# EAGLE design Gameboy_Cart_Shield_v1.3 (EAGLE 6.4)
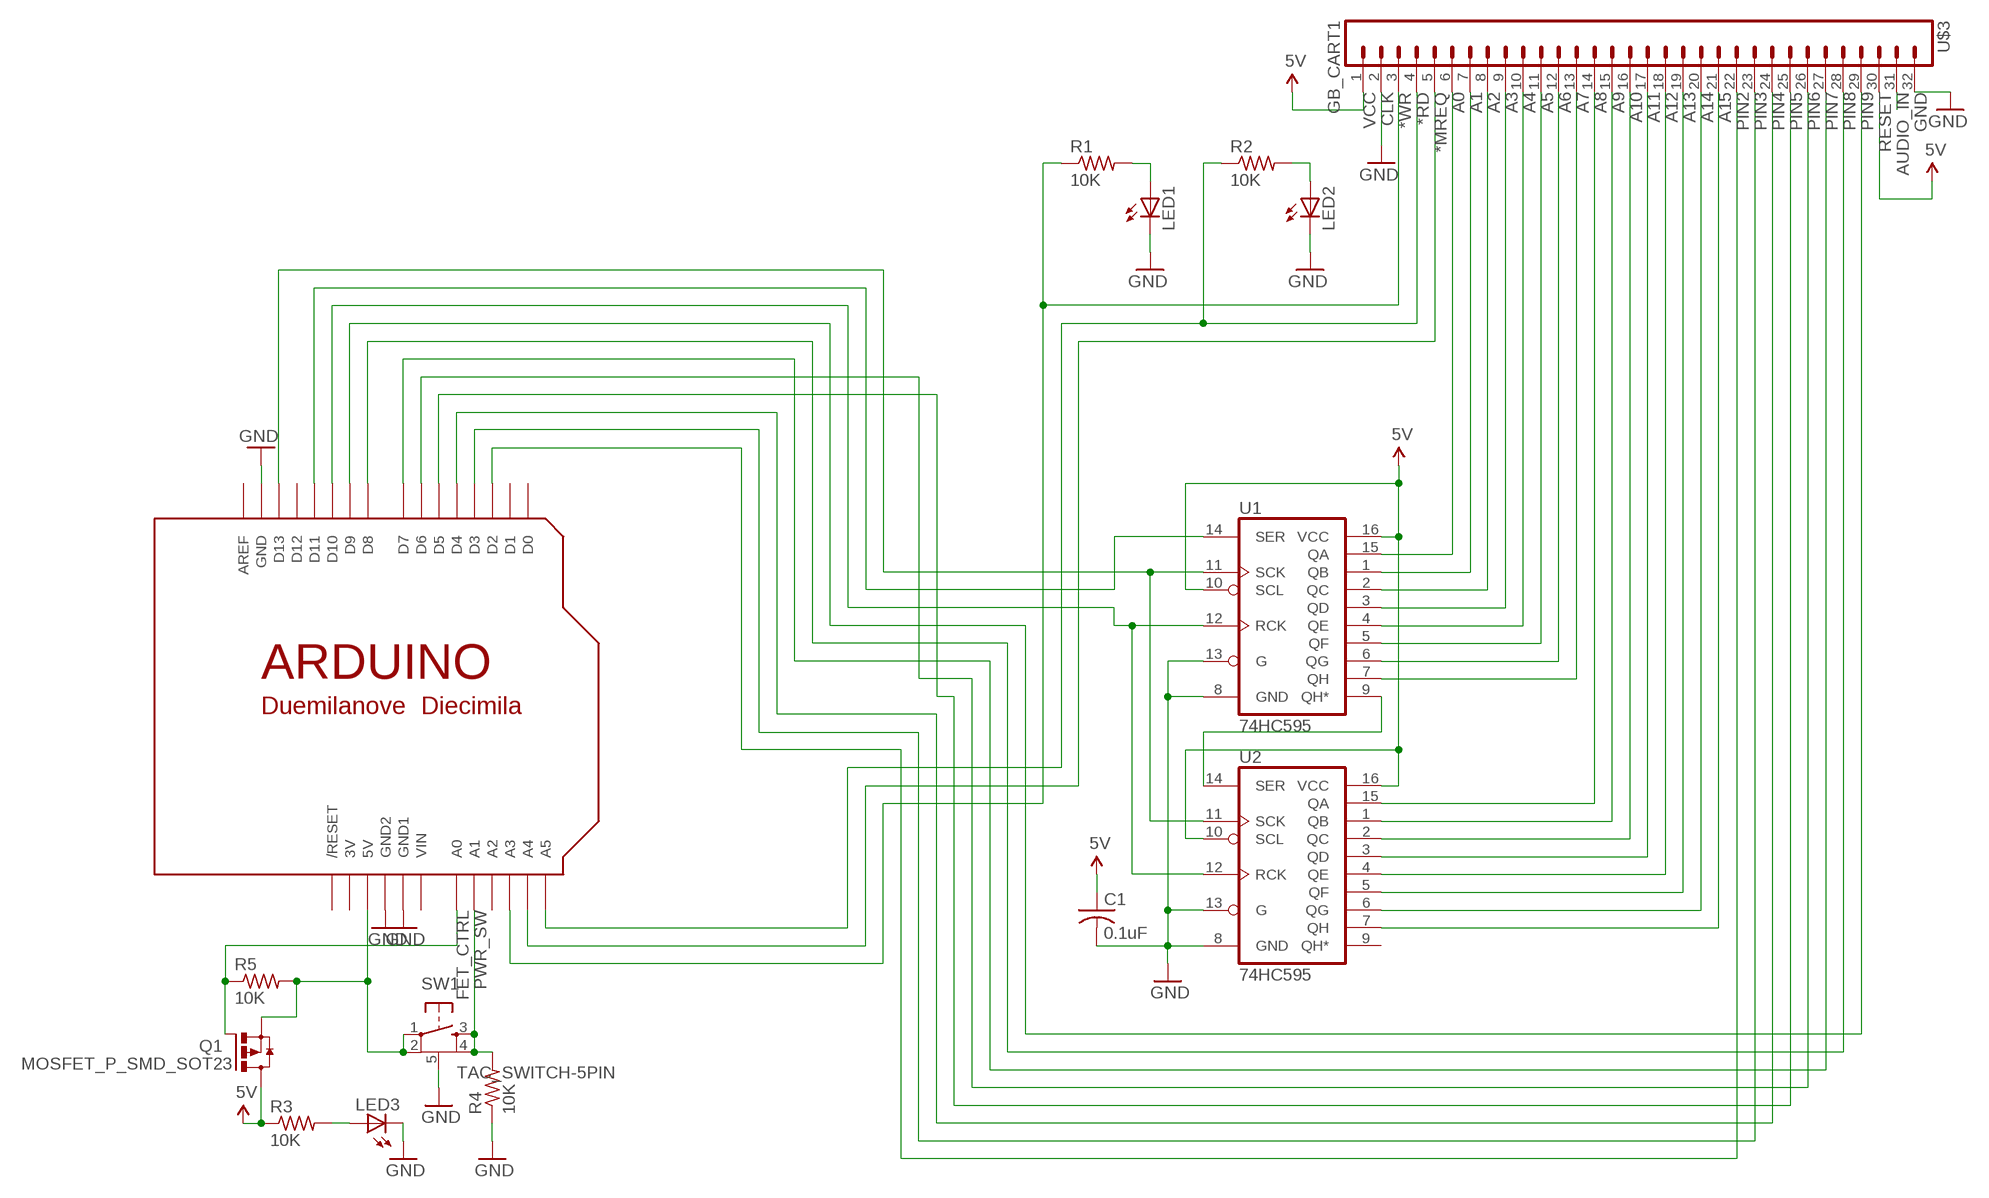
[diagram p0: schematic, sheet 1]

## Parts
C1  0.1uF  C-USC0805K  [C0805K]
LED1  LEDCHIP-LED0805  [CHIP-LED0805]
LED2  LEDCHIP-LED0805  [CHIP-LED0805]
LED3  LEDCHIP-LED0805  [CHIP-LED0805]
Q1  MOSFET_P_SMD_SOT23  [SUPER-SOT3]
R1  10K  R-US_R0805_2  [R0805_2]
R2  10K  R-US_R0805_2  [R0805_2]
R3  10K  R-US_R0805_2  [R0805_2]
R4  10K  R-US_R0805_2  [R0805_2]
R5  10K  R-US_R0805_2  [R0805_2]
SW1  TAC_SWITCH-5PIN  [TACTILE_SWITCH_SMD_6MM]
U1  74HC595  74LS595D  [SO16]
U2  74HC595  74LS595D  [SO16]
U$1  ARDUINONODIMA  [ARDUINO-NODIMA]
U$3  GB_CART1  [GB_CART_1]

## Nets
*MREQ: U$1.A4 U$3.5
*RD: R2.1 U$1.A5 U$3.4
*WR: R1.1 U$1.A3 U$3.3
A0: U1.15(QA) U$3.6
A1: U1.1(QB) U$3.7
A2: U1.2(QC) U$3.8
A3: U1.3(QD) U$3.9
A4: U1.4(QE) U$3.10
A5: U1.5(QF) U$3.11
A6: U1.6(QG) U$3.12
A7: U1.7(QH) U$3.13
A8: U2.15(QA) U$3.14
A9: U2.1(QB) U$3.15
A10: U2.2(QC) U$3.16
A11: U2.3(QD) U$3.17
A12: U2.4(QE) U$3.18
A13: U2.5(QF) U$3.19
A14: U2.6(QG) U$3.20
A15: U2.7(QH) U$3.21
AUDIO_IN: U$3.31
FET_CTRL: Q1.1(G) R5.1 U$1.A0
GND: C1.2 LED1.C LED2.C LED3.C R4.1 SW1.5 U1.8(GND) U1.13(G) U2.8(GND) U2.13(G) U$1.GND U$1.GND1 U$1.GND2 U$3.2 U$3.32
N$1: LED2.A R2.2
N$2: LED3.A R3.2
N$6: LED1.A R1.2
N$7: Q1.2(S) R5.2 SW1.1 SW1.2 U$1.5V
N$10: U1.9(QH*) U2.14(SER)
PIN2: U$1.D2 U$3.22
PIN3: U$1.D3 U$3.23
PIN4: U$1.D4 U$3.24
PIN5: U$1.D5 U$3.25
PIN6: U$1.D6 U$3.26
PIN7: U$1.D7 U$3.27
PIN8: U$1.D8 U$3.28
PIN9: U$1.D9 U$3.29
PIN10: U1.12(RCK) U2.12(RCK) U$1.D10
PIN11: U1.14(SER) U$1.D11
PIN12: U1.11(SCK) U2.11(SCK) U$1.D13
PWR_SW: R4.2 SW1.3 SW1.4 U$1.A1
VCC: C1.1 Q1.3(D) R3.1 U1.10(SCL) U1.16(VCC) U2.10(SCL) U2.16(VCC) U$3.1 U$3.30 ; supply symbol labelled 5V
Unconnected: U2.9(QH*) U$1.A2 U$1.AREF U$1.D0 U$1.D1 U$1.D12 U$1.RESET(/RESET)

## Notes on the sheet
- VCC | CLK | RESET

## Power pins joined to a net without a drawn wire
3V: U$1.3V
VIN: U$1.VIN

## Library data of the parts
C1 = adafruit:C-US: CAPACITOR, American symbol
LED1-LED3 = adafruit:LED: LED
Q1 = transistor-power_old:MOSFET_P_SMD_SOT23
R1-R5 = adafruit:R-US_: RESISTOR, American symbol
SW1 = SparkFun:TAC_SWITCH-5PIN
U1 U2 = SparkFun:74*595: 8-bit SHIFT REGISTER, output latch
U$1 = adafruit:ARDUINO: Arduino Diecimila/Duemilanove Make a shield with ease, this package has all the named pins as well as the two mounting drill holes and an outline of the USB and DC power connector. The outline is on the DIMENSION layer, so if your board house uses it they will cut the outline to match.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
U$3 = alex:GB_CART

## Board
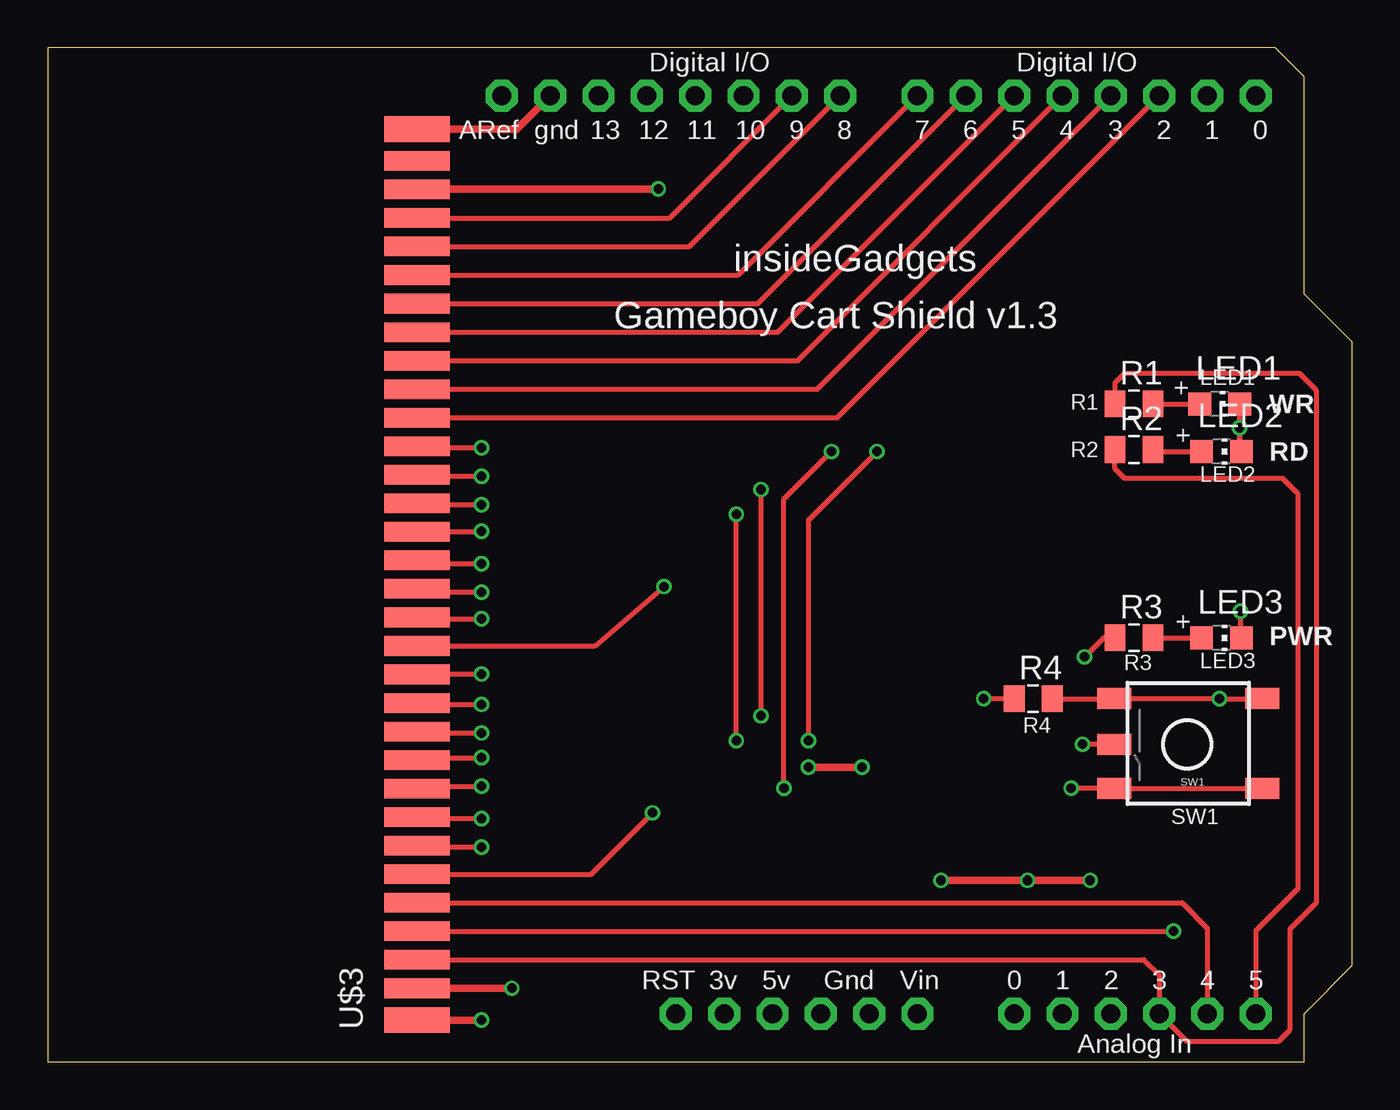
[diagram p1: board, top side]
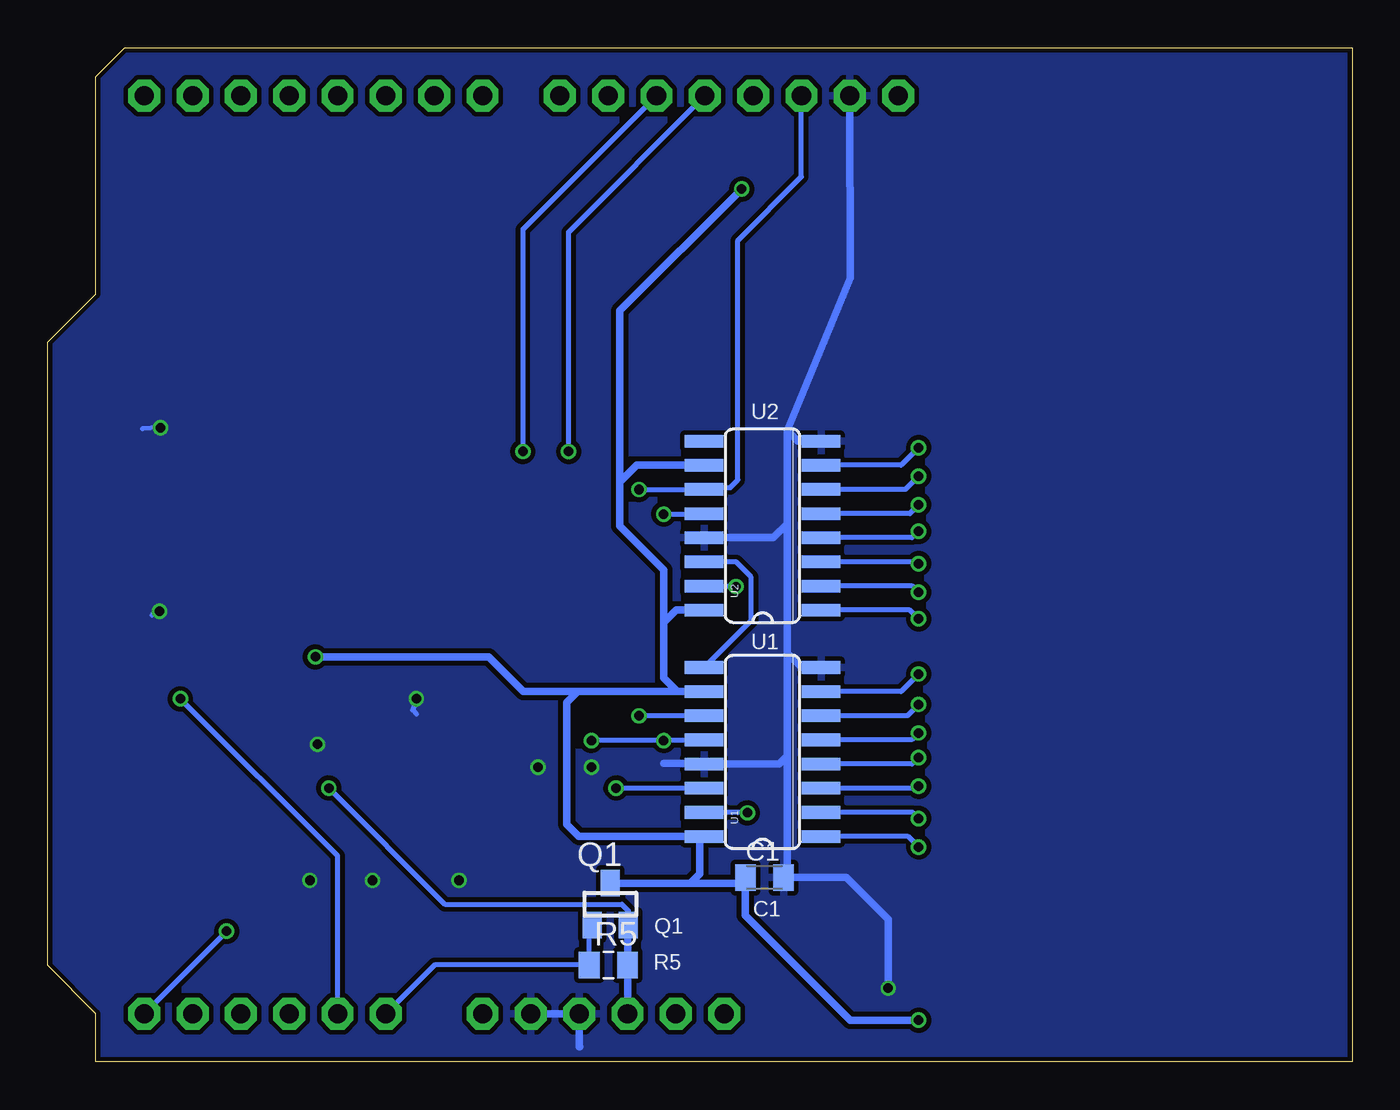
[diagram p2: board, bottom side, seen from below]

Size 68.58 x 53.34 mm. Coordinates in mm from the lower left corner, seen from the top.
Copper layers (1*16): Top 0.035mm / dielectric 1.5mm / Bottom 0.035mm
Design rules "ITEADstudio_DRC": minimum track width 6mil, minimum drill 12mil, track to track 6mil, track to pad 6mil, pad to pad 6mil, via to via 6mil, smd to smd 0mil, copper to edge 10mil, drill to drill 10mil, minimum pad ring 10mil, minimum via ring 6mil, stop-mask expansion 2mil, vias tented up to drill 100mil, thermal gap 10mil

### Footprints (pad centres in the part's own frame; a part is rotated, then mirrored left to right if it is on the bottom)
C0805K = smd 1.1 x 1.4: 1 -1,0; 2 1,0
CHIP-LED0805 = smd 1.2 x 1.2: A 0,-1.05; C 0,1.05
SUPER-SOT3 = smd 1 x 1.4: 1 -0.95,-1.1; 2 0.95,-1.1; 3 0,1.1
R0805_2 = smd 1.1 x 1.4: 1 -1,0; 2 1,0
TACTILE_SWITCH_SMD_6MM = smd 1.8 x 1.1: 1 -4.54,1.705; 2 3.24,1.705; 3 -4.54,-3.005; 4 3.24,-3.005; 5 3.24,-0.595
SO16 = smd 0.66 x 2.032: 1 -4.445,-3.073; 2 -3.175,-3.073; 3 -1.905,-3.073; 4 -0.635,-3.073; 5 0.635,-3.073; 6 1.905,-3.073; 7 3.175,-3.073; 8 4.445,-3.073; 9 4.445,3.073; 10 3.175,3.073; 11 1.905,3.073; 12 0.635,3.073; 13 -0.635,3.073; 14 -1.905,3.073; 15 -3.175,3.073; 16 -4.445,3.073
ARDUINO-NODIMA = drill 1 pad 1.676 octagon: 3V 35.56,2.54; 5V 38.1,2.54; A0 50.8,2.54; A1 53.34,2.54; A2 55.88,2.54; A3 58.42,2.54; A4 60.96,2.54; A5 63.5,2.54; AREF 23.876,50.8; D0 63.5,50.8; D1 60.96,50.8; D2 58.42,50.8; D3 55.88,50.8; D4 53.34,50.8; D5 50.8,50.8; D6 48.26,50.8; D7 45.72,50.8; D8 41.656,50.8; D9 39.116,50.8; D10 36.576,50.8; D11 34.036,50.8; D12 31.496,50.8; D13 28.956,50.8; GND 26.416,50.8; GND1 43.18,2.54; GND2 40.64,2.54; RESET 33.02,2.54; VIN 45.72,2.54
GB_CART_1 = smd 1.36 x 3.46: 1 -22.895,-0.12; 32 23.94,-0.12 | smd 1.03 x 3.46: 2 -21.225,-0.12; 3 -19.725,-0.12; 4 -18.225,-0.12; 5 -16.725,-0.12; 6 -15.225,-0.12; 7 -13.725,-0.12; 8 -12.225,-0.12; 9 -10.725,-0.12; 10 -9.225,-0.12; 11 -7.725,-0.12; 12 -6.225,-0.12; 13 -4.725,-0.12; 14 -3.225,-0.12; 15 -1.725,-0.12; 16 -0.225,-0.12; 17 1.275,-0.12; 18 2.775,-0.12; 19 4.275,-0.12; 20 5.775,-0.12; 21 7.275,-0.12; 22 8.775,-0.12; 23 10.275,-0.12; 24 11.775,-0.12; 25 13.275,-0.12; 26 14.775,-0.12; 27 16.275,-0.12; 28 17.775,-0.12; 29 19.275,-0.12; 30 20.775,-0.12; 31 22.275,-0.12

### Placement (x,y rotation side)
C1  30.9,9.7 0 bottom
LED1  61.6,34.6 270 top
LED2  61.7,32.1 270 top
LED3  61.7,22.3 270 top
Q1  39,8.3 0 bottom
R1  57.1,34.6 0 top
R2  57.1,32.2 0 top
R3  57.1,22.3 0 top
R4  51.8,19.1 0 top
R5  39.1,5.1 0 bottom
SW1  59.3,16.1 180 top
U1  31,16.3 90 bottom
U2  31,28.2 90 bottom
U$1  0,0 0 top
U$3  19.3,25.1 90 top

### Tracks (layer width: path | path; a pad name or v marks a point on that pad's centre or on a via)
*MREQ
  Top 0.254: U$3.5 59.62,8.38 60.96,7.04 U$1.A4
*RD  (via drill 0.5)
  Top 0.254: 19.42,6.9 U$3.4 v59.17,6.88 | R2.1 56.1,31.2 56.6,30.7 64.9,30.7 65.7,29.9 65.7,9.1 63.5,6.9 U$1.A5
  Bottom 0.254: v59.17,6.88 59.16,6.88 U$1.A5
*WR
  Top 0.254: U$3.3 57.62,5.38 58.42,4.58 U$1.A3 59.86,1.1 64.7,1.1 65.3,1.7 65.3,7 66.7,8.4 66.7,35.3 65.8,36.2 56.6,36.2 56.1,35.7 R1.1
A0  (via drill 0.5)
  Top 0.254: v31.8,13.1 28.58,9.88 U$3.6
  Bottom 0.254: v31.8,13.1 31.83,13.13 U1.15
A1  (via drill 0.5)
  Top 0.254: U$3.7 19.49,11.3 v22.8,11.3
  Bottom 0.254: U1.1 23.36,11.86 v22.8,11.3
A2  (via drill 0.5)
  Top 0.254: U$3.8 19.49,12.8 v22.8,12.8
  Bottom 0.254: v22.8,12.8 23.12,13.13 U1.2
A3  (via drill 0.5)
  Top 0.254: U$3.9 19.55,14.5 v22.8,14.5
  Bottom 0.254: U1.3 22.91,14.4 v22.8,14.5
A4  (via drill 0.5)
  Top 0.254: v22.8,16 19.55,16 U$3.10
  Bottom 0.254: U1.4 23.13,15.67 v22.8,16
A5  (via drill 0.5)
  Top 0.254: v22.8,17.3 19.49,17.3 U$3.11
  Bottom 0.254: U1.5 23.16,16.94 v22.8,17.3
A6  (via drill 0.5)
  Top 0.254: v22.8,18.8 19.49,18.8 U$3.12
  Bottom 0.254: U1.6 23.39,18.21 v22.8,18.8
A7  (via drill 0.5)
  Top 0.254: v22.8,20.4 19.44,20.4 U$3.13
  Bottom 0.254: U1.7 23.72,19.48 v22.8,20.4
A8  (via drill 0.5)
  Top 0.254: v32.4,25 28.77,21.88 U$3.14
  Bottom 0.254: v32.4,25 34.05,25 U2.15
A9  (via drill 0.5)
  Top 0.254: v22.8,23.3 19.49,23.3 U$3.15
  Bottom 0.254: U2.1 23.25,23.76 v22.8,23.3
A10  (via drill 0.5)
  Top 0.254: v22.8,24.7 19.59,24.7 U$3.16
  Bottom 0.254: U2.2 23.12,25.03 v22.8,24.7
A11  (via drill 0.5)
  Top 0.254: v22.8,26.2 19.59,26.2 U$3.17
  Bottom 0.254: U2.3 22.89,26.3 v22.8,26.2
A12  (via drill 0.5)
  Top 0.254: v22.8,27.9 19.44,27.9 U$3.18
  Bottom 0.254: U2.4 23.13,27.57 v22.8,27.9
A13  (via drill 0.5)
  Top 0.254: v22.8,29.3 19.49,29.3 U$3.19
  Bottom 0.254: U2.5 23.27,28.84 v22.8,29.3
A14  (via drill 0.5)
  Top 0.254: v22.8,30.8 19.49,30.8 U$3.20
  Bottom 0.254: U2.6 23.49,30.11 v22.8,30.8
A15  (via drill 0.5)
  Top 0.254: v22.8,32.3 19.49,32.3 U$3.21
  Bottom 0.254: U2.7 23.72,31.38 v22.8,32.3
FET_CTRL
  Bottom 0.254: Q1.1 40.1,7.05 R5.1 48.24,5.1 U$1.A0
GND  (via drill 0.5)
  Top 0.254: R4.1 v49.2,19.1 | SW1.5 54.61,16.7 v54.4,16.7 | LED3.C 62.7,22.35 v62.7,23.7 | LED2.C 62.65,32.2 v62.65,33.35 | v62.65,33.35 LED1.C | LED2.C 62.7,32.25 | v62.65,33.35 62.65,32.1 LED2.C
  Top 0.406: U$3.32 24.66,49.04 U$1.GND | U$3.2 v24.4,3.88 | v40,15.5 v42.8,15.5 | v46.95,9.55 v51.5,9.55 v54.8,9.55
  Bottom 0.254: U2.8 27.98,32.7 | U1.13 34.07,15.7 | v49.2,19.1 49.4,18.5 49.2,18.3 | v54.4,16.7 54.2,16.7 54.1,16.8 | v62.7,23.7 63.1,23.5 | v62.65,33.35 63.6,33.3
  Bottom 0.406: U2.13 30.44,27.57 29.7,28.3 | U1.13 30.13,15.67 29.7,16.1 | 29.7,21.5 29.7,16.1 | 29.7,21.5 29.7,28.3 | U1.8 28.94,20.75 29.7,21.5 | 29.7,28.3 29.7,33.2 | 29.7,33.2 26.4,41.22 U$1.GND | 34.07,15.7 36.2,15.7 | U2.8 29.14,32.65 29.7,33.2 | v24.4,3.88 24.4,7.5 26.6,9.7 C1.2 29.7,9.9 29.7,16.1 | U$1.GND1 U$1.GND2 40.64,0.8 40.6,0.8
  pour Bottom (isolate 0.254): -2.5,55.5 73.2,55.5 73.2,-9.9 -2.5,-9.9
N$1
  Top 0.254: LED2.A 58,32.1 R2.2
N$2
  Top 0.254: R3.2 LED3.A
N$6
  Top 0.254: R1.2 LED1.A
N$7  (via drill 0.5)
  Top 0.254: v53.8,14.4 SW1.2 SW1.1
  Bottom 0.254: 38.1,7.15 Q1.2 38.05,7.95 38.4,8.3 47.7,8.3 v53.8,14.4
  Bottom 0.406: 38.1,7.15 R5.2 U$1.5V
N$10
  Bottom 0.254: U1.9 31.6,23.22 31.6,25.5 32.39,26.3 U2.14
PIN2
  Top 0.254: U$1.D2 41.49,33.88 U$3.22
PIN3
  Top 0.254: U$1.D3 40.45,35.38 U$3.23
PIN4
  Top 0.254: U$1.D4 39.41,36.88 U$3.24
PIN5
  Top 0.254: U$1.D5 38.38,38.38 U$3.25
PIN6
  Top 0.254: U$1.D6 37.33,39.88 U$3.26
PIN7
  Top 0.254: U$1.D7 36.3,41.38 U$3.27
PIN8
  Top 0.254: U$1.D8 33.73,42.88 U$3.28
PIN9
  Top 0.254: U$1.D9 32.69,44.38 U$3.29
PIN10  (via drill 0.5)
  Top 0.254: v36.2,16.9 v36.2,28.8 | v40,16.9 40,28.5 v43.6,32.1
  Bottom 0.254: U2.12 34.11,28.8 v36.2,28.8 | U1.12 34.11,16.9 v36.2,16.9 v40,16.9 | U$1.D10 43.6,43.78 v43.6,32.1
PIN11  (via drill 0.5)
  Top 0.254: v38.7,14.4 38.7,29.6 v41.2,32.1
  Bottom 0.254: U1.14 38.99,14.4 v38.7,14.4 | U$1.D11 41.2,43.64 v41.2,32.1
PIN12  (via drill 0.5)
  Top 0.254: v37.5,18.2 v37.5,30.1
  Bottom 0.254: v37.5,30.1 34.27,30.1 34.17,30.2 U2.11 33.98,30.2 32.7,30.2 32.3,30.6 32.3,43.2 28.96,46.54 U$1.D13 | U1.11 v37.5,18.2
PWR_SW  (via drill 0.5)
  Top 0.254: SW1.3 v61.6,19.1 v61.6,19.11 SW1.4 R4.2
  Bottom 0.254: U$1.A1 53.34,10.84 v61.6,19.1
VCC  (via drill 0.5)
  Top 0.254: 19.44,45.9 U$3.30 | U$3.1 | R3.1 55.5,22.3 v54.5,21.3
  Top 0.406: U$3.1 v22.8,2.2 | 19.44,45.9 v32.1,45.9
  Bottom 0.254: U2.16 34.12,23.8 | 34.22,12 U1.16 34.3,11.63
  Bottom 0.406: 40.72,19.48 U1.10 | 40.72,19.48 41.3,18.9 41.3,12.5 40.66,11.86 U1.16 | 34.3,11.63 34.3,9.9 34.8,9.4 | Q1.3 35.4,9.4 34.8,9.4 | v54.5,21.3 45.4,21.3 43.58,19.48 40.72,19.48 | 35.08,19.48 U1.10 | U1.10 35.47,19.48 36.2,20.2 36.2,23.1 | v32.1,45.9 38.5,39.5 38.5,30.5 | 38.5,30.5 38.5,28.18 36.2,25.88 36.2,23.1 | U2.10 37.62,31.38 38.5,30.5 | U2.16 35.55,23.76 36.2,23.1 | v22.8,2.2 26.4,2.2 31.9,7.7 C1.1 32.2,9.4 34.8,9.4

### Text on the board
_tsilk: insideGadgets | Gameboy Cart Shield v1.3 | LED1 | R1 | WR | R2 | RD | LED2 | PWR | LED3 | R3 | R4 | SW1
_bsilk: U2 | U1 | C1 | Q1 | R5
